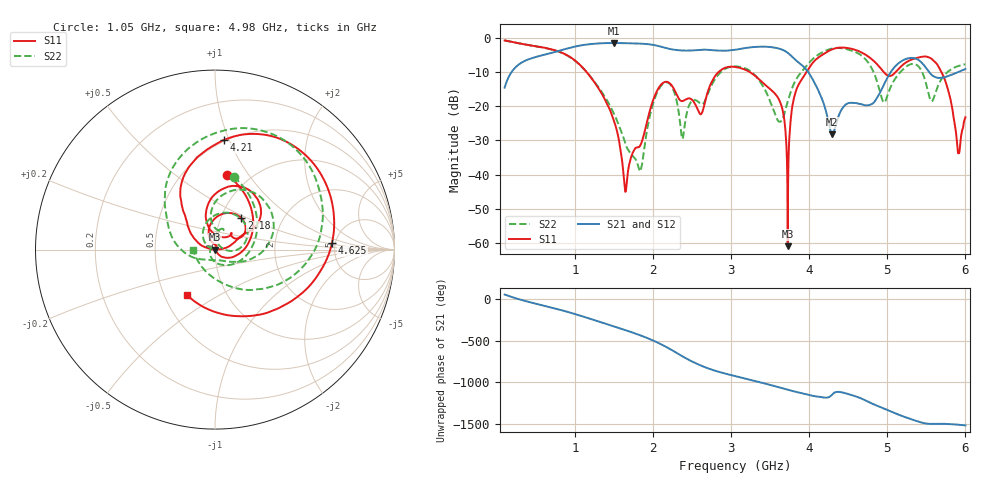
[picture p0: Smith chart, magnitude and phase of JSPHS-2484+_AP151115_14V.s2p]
!Mini-Circuits Laboratory
!S-Parameters
!Run/Lot/Date Code:MF33450/NA/1551
!Fixture/SN/Due: 90-4-20-21/70546/03/17/16
!Connection:PORT<IN> - pin<1>; PORT<OUT> - pin<7>;PORT<BIAS> - pin<4>;
!Tested With:PORT EXTENTION
!Network Analyzer:AG E5071C/74883/05/12/16
!Created: 01-07-2016 at 14:11:25
!MODEL: JSPHS-2484+
!S/N: V=14V
# MHZ S DB R 50
!Frequency  S11 dB  S11 DEG  S21 dB  S21 DEG  S12 dB  S12 DEG  S22 dB  S22 DEG
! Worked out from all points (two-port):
!   1181 points, 100 MHz to 6 GHz, reference 50 ohm
!   highest |S21| = -1.42 dB at 1.5 GHz (marker M1); lowest = -28.2 dB at 4.295 GHz (marker M2)
!   |S21| within 3 dB of the highest: 686.8 MHz to 3.733 GHz (3.046 GHz wide, 138 % of centre)
!   lowest |S11| = -61.0 dB at 3.725 GHz (marker M3), VSWR 1.00, Z = 50.1 + j0.0171 ohm
!   |S11| at or under -10 dB: 1.152 GHz to 2.837 GHz (1.685 GHz wide, 84.5 % of centre); 3.244 GHz to 3.963 GHz (719.1 MHz wide, 20 % of centre); 5.696 GHz to end of sweep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
!   |S22| runs from -39.1 to -0.7 dB; largest |S21 - S12| = 0.0022
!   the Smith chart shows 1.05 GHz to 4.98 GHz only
!   S11 on the Smith chart (normalised r, x): 1.05 GHz: 0.78, +0.79; 2.18 GHz: 1.25, +0.46; 4.21 GHz: 0.49, +0.95; 4.625 GHz: 4.69, +0.58; 4.98 GHz: 0.65, -0.36
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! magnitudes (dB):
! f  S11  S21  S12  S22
! 100 MHz  -0.7  -14.5  -14.5  -0.7
! 1.05 GHz  -7.5  -2.2  -2.2  -7.6
! 1.085 GHz  -8.3  -2.1  -2.1  -8.3
! 1.5 GHz  -24.3  -1.4  -1.4  -22.1
! 1.65 GHz  -45.0  -1.5  -1.5  -31.2
! 1.84 GHz  -31.3  -1.6  -1.6  -39.1
! 2.07 GHz  -14.7  -2.3  -2.3  -15.2
! 2.18 GHz  -12.8  -3.0  -3.0  -13.0
! 2.38 GHz  -18.4  -3.6  -3.6  -29.5
! 3.05 GHz  -8.4  -3.4  -3.4  -8.2
! 3.605 GHz  -17.6  -3.0  -3.0  -24.3
! 3.725 GHz  -61.0  -4.3  -4.3  -18.6
! 3.81 GHz  -17.1  -6.0  -6.1  -13.1
! 4.035 GHz  -7.5  -11.7  -11.6  -6.3
! 4.21 GHz  -4.3  -21.0  -21.2  -3.7
! 4.295 GHz  -3.3  -28.2  -28.1  -3.0
! 4.625 GHz  -3.7  -19.2  -19.3  -4.4
! 4.98 GHz  -10.5  -12.5  -12.5  -18.3
! 5.02 GHz  -11.1  -10.8  -10.8  -15.6
! 5.55 GHz  -5.8  -10.3  -10.3  -18.0
! 5.91 GHz  -33.8  -9.9  -9.9  -8.2
! 6 GHz  -23.2  -9.0  -9.0  -7.6
